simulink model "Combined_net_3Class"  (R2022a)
settings: Solver=FixedStepAuto  StartTime=0.0  StopTime=simtime  FixedStep=1  RelTol=1e-3
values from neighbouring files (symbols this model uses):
  simtime = length(SOC_CC{1, 1})    [Data_preparation.m]    (also in SimulationCycle.m = cell2mat(simtime_og(i)))
  SOH_predict = double(ans.SOHout(simtime))    [SimulationCycle.m]
undefined symbols (not defined in the file or in its folder): dSOC_mu_CC, dSOC_sig_CC, dv_mu_CC, dv_sig_CC, SOC_mu_CC, SOC_sig_CC, SOE_mu_CC, SOE_sig_CC
libraries: neural x121, deeplib x1
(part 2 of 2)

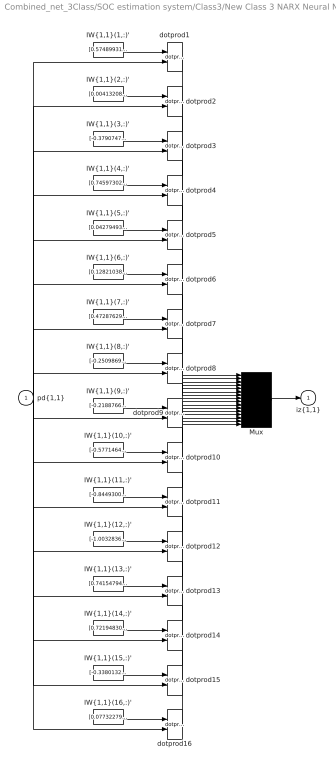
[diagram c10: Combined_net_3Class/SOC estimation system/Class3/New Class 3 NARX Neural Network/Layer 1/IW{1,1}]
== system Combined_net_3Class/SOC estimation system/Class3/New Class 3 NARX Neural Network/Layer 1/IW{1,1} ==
  "pd{1,1}" : Inport  PortDimensions=6  SampleTime=1
  "IW{1,1}(1,:)'" : Constant  Value=[0.57489931629684110081512926626601256430149078369140625;-0.3515011151766405106400270597077906131744384765625;-0.235240138064670478712514523067511618137359619140625;-0.415665695112699740132455872299033217132091522216796875;-0.54083277905494309134581953912856988608837127685546875;0.2491902947301962989445911489383433945477008819580078125]
  "IW{1,1}(10,:)'" : Constant  Value=[-0.57714648597659190532027650988311506807804107666015625;0.047702980401234530705156799967880942858755588531494140625;0.438905821704081822165477433372871018946170806884765625;0.5136719729138483625519029374117963016033172607421875;-0.06710567452929290521712601957915467210114002227783203125;-0.451124189798159325182069778747973032295703887939453125]
  "IW{1,1}(11,:)'" : Constant  Value=[-0.84493007670864195279847308484022505581378936767578125;0.0299673301415608085707109609074905165471136569976806640625;0.63504695757984752635394443132099695503711700439453125;-0.78817262284074451894611001989687792956829071044921875;0.91885523230133447913914324090001173317432403564453125;-0.8192881318045144301009941045776940882205963134765625]
  "IW{1,1}(12,:)'" : Constant  Value=[-1.00328365957425713617112705833278596401214599609375;-0.4162739419152441389115892889094538986682891845703125;0.2778056257659071714982701450935564935207366943359375;0.81259865037192724468440019336412660777568817138671875;1.23650985871420449058177837287075817584991455078125;-0.2929172509986999184405931373476050794124603271484375]
  "IW{1,1}(13,:)'" : Constant  Value=[0.74154794238423249463920683410833589732646942138671875;-0.48527842225931550057538288456271402537822723388671875;0.86708245679925510795982290801475755870342254638671875;-0.1759789359971944133764765183514100499451160430908203125;-1.3752493967582399836402373693999834358692169189453125;-0.00091260160326845523627581346914894311339594423770904541015625]
  "IW{1,1}(14,:)'" : Constant  Value=[0.72194830081038130487058879225514829158782958984375;0.083263215679716839900947888963855803012847900390625;0.768923477287991818940326993470080196857452392578125;0.1933662663322287811329402984483749605715274810791015625;1.308738303825084159370817360468208789825439453125;-0.57527297822178213859700690591125749051570892333984375]
  "IW{1,1}(15,:)'" : Constant  Value=[-0.338013217203540328181787799621815793216228485107421875;-0.11116352190086421780623737731730216182768344879150390625;-0.636515796112465448430839387583546340465545654296875;-1.03325458248108947856280792620964348316192626953125;1.334039636242204007743339388980530202388763427734375;0.93930340463265993289354582884698174893856048583984375]
  "IW{1,1}(16,:)'" : Constant  Value=[0.07732279602847856592173769740838906727731227874755859375;-0.406242406915276077494780793131212703883647918701171875;0.0246450504641358043855792203657983918674290180206298828125;-0.07305262802981961345327732715304591692984104156494140625;0.38838168508634407505297758689266629517078399658203125;-0.02468603065919001970929258504838799126446247100830078125]
  "IW{1,1}(2,:)'" : Constant  Value=[0.004132082293141054428475822390964822261594235897064208984375;-0.07626335722691372775994267385613056831061840057373046875;0.012693474527892857628419420734644518233835697174072265625;-0.0058209828312985149867397893785891938023269176483154296875;0.0780918658530748988066960691867279820144176483154296875;-0.01319417224404989714969804737165759433992207050323486328125]
  "IW{1,1}(3,:)'" : Constant  Value=[-0.379074783991779185043924371711909770965576171875;1.016745025307583372153885648003779351711273193359375;-0.442564886903998366829426913682254962623119354248046875;0.93193801751100113772707800308126024901866912841796875;-0.54900708871000547528495872029452584683895111083984375;0.56770819572392994256659903840045444667339324951171875]
  "IW{1,1}(4,:)'" : Constant  Value=[0.745973028967485074502974384813569486141204833984375;0.76493541460268821285950480159954167902469635009765625;-0.68912609389738832543770286065409891307353973388671875;0.07391887270039194934856396912437048740684986114501953125;0.81792600024676165304526875843293964862823486328125;0.27949425616045697751133047859184443950653076171875]
  "IW{1,1}(5,:)'" : Constant  Value=[0.04279493192384183075649417560271103866398334503173828125;-0.24990879501025708986361451025004498660564422607421875;0.008266010129701496789156323075076215900480747222900390625;-0.03680818383380424219097903915098868310451507568359375;0.225757554997183917944170161717920564115047454833984375;-0.008529510970860222640599346277667791582643985748291015625]
  "IW{1,1}(6,:)'" : Constant  Value=[0.12821038490724101510664922898286022245883941650390625;-0.58355828505747309176143744480214081704616546630859375;0.005953497815920946560630522270685105468146502971649169921875;-0.111167669930111123743898815519060008227825164794921875;0.52302756879668221845491871135891415178775787353515625;-0.00612713488324014531050121235011829412542283535003662109375]
  "IW{1,1}(7,:)'" : Constant  Value=[0.472876296890176905929337181078153662383556365966796875;0.507349771020651818531632670783437788486480712890625;0.4316557440097958942004652271862141788005828857421875;-0.58380532843848154112009751770528964698314666748046875;-0.0755903965904468899683621430085622705519199371337890625;-0.447270650721935447702293231486692093312740325927734375]
  "IW{1,1}(8,:)'" : Constant  Value=[-0.2509869071349084546085350666544400155544281005859375;0.341748594182761544768567318897112272679805755615234375;-0.6811569018579881618080662519787438213825225830078125;-0.98272991511463125835490473036770708858966827392578125;-0.82930046363700693490272897179238498210906982421875;0.60682317912345029586873579319217242300510406494140625]
  "IW{1,1}(9,:)'" : Constant  Value=[-0.2188766968978141658208613762326422147452831268310546875;-0.4951250680687657723666461606626398861408233642578125;-0.3781747939072890307699026379850693047046661376953125;0.51581894069656220036534932660288177430629730224609375;-0.53936529448250791762831113373977132141590118408203125;0.348952666019013424403283352148719131946563720703125]
  Mux : Mux  Inputs=16
  dotprod{1..16} (16 alike) : neural/Weight Functions/dotprod
  "iz{1,1}" : Outport
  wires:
  "IW{1,1}(1,:)'"/1 -> dotprod1/1
  "pd{1,1}"/1 -> dotprod1/2, dotprod2/2, dotprod3/2, dotprod4/2, dotprod5/2, dotprod6/2, dotprod7/2, dotprod8/2, dotprod9/2, dotprod10/2, dotprod11/2, dotprod12/2, dotprod13/2, dotprod14/2, dotprod15/2, dotprod16/2
  dotprod1/1 -> Mux/1
  "IW{1,1}(2,:)'"/1 -> dotprod2/1
  dotprod2/1 -> Mux/2
  "IW{1,1}(3,:)'"/1 -> dotprod3/1
  dotprod3/1 -> Mux/3
  "IW{1,1}(4,:)'"/1 -> dotprod4/1
  dotprod4/1 -> Mux/4
  "IW{1,1}(5,:)'"/1 -> dotprod5/1
  dotprod5/1 -> Mux/5
  "IW{1,1}(6,:)'"/1 -> dotprod6/1
  dotprod6/1 -> Mux/6
  "IW{1,1}(7,:)'"/1 -> dotprod7/1
  dotprod7/1 -> Mux/7
  "IW{1,1}(8,:)'"/1 -> dotprod8/1
  dotprod8/1 -> Mux/8
  "IW{1,1}(9,:)'"/1 -> dotprod9/1
  dotprod9/1 -> Mux/9
  "IW{1,1}(10,:)'"/1 -> dotprod10/1
  dotprod10/1 -> Mux/10
  "IW{1,1}(11,:)'"/1 -> dotprod11/1
  dotprod11/1 -> Mux/11
  "IW{1,1}(12,:)'"/1 -> dotprod12/1
  dotprod12/1 -> Mux/12
  "IW{1,1}(13,:)'"/1 -> dotprod13/1
  dotprod13/1 -> Mux/13
  "IW{1,1}(14,:)'"/1 -> dotprod14/1
  dotprod14/1 -> Mux/14
  "IW{1,1}(15,:)'"/1 -> dotprod15/1
  dotprod15/1 -> Mux/15
  "IW{1,1}(16,:)'"/1 -> dotprod16/1
  dotprod16/1 -> Mux/16
  Mux/1 -> "iz{1,1}"/1

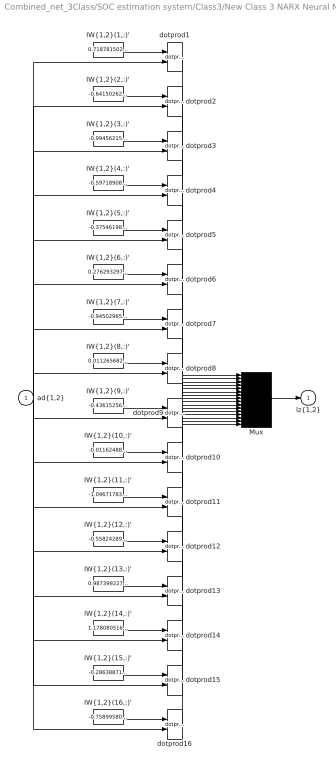
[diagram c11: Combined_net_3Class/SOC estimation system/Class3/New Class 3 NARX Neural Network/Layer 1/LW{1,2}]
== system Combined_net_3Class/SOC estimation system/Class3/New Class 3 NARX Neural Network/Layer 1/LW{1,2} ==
  "ad{1,2}" : Inport  PortDimensions=1  SampleTime=1
  "IW{1,2}(1,:)'" : Constant  Value=0.71878150211169489214313443881110288202762603759765625
  "IW{1,2}(10,:)'" : Constant  Value=-0.01162488589042467122813828694916082895360887050628662109375
  "IW{1,2}(11,:)'" : Constant  Value=-1.0967178319018591192701705949730239808559417724609375
  "IW{1,2}(12,:)'" : Constant  Value=-0.55824289911548652387551783249364234507083892822265625
  "IW{1,2}(13,:)'" : Constant  Value=0.9873992270040805596664768017944879829883575439453125
  "IW{1,2}(14,:)'" : Constant  Value=1.1780805168430548146574210477410815656185150146484375
  "IW{1,2}(15,:)'" : Constant  Value=-0.28638871201418203416011465378687717020511627197265625
  "IW{1,2}(16,:)'" : Constant  Value=-0.758995805205835427642568902228958904743194580078125
  "IW{1,2}(2,:)'" : Constant  Value=-0.64150262074499320164022719836793839931488037109375
  "IW{1,2}(3,:)'" : Constant  Value=-0.9945621582289432272006024504662491381168365478515625
  "IW{1,2}(4,:)'" : Constant  Value=-0.59718908368235179562333314606803469359874725341796875
  "IW{1,2}(5,:)'" : Constant  Value=-0.37546198082295989539858283023932017385959625244140625
  "IW{1,2}(6,:)'" : Constant  Value=0.276293297318553732200285821818397380411624908447265625
  "IW{1,2}(7,:)'" : Constant  Value=-0.9450296512095632817107571099768392741680145263671875
  "IW{1,2}(8,:)'" : Constant  Value=0.01126568217795320507590428604771659593097865581512451171875
  "IW{1,2}(9,:)'" : Constant  Value=-0.436152569616356677872914815452531911432743072509765625
  Mux : Mux  Inputs=16
  dotprod{1..16} (16 alike) : neural/Weight Functions/dotprod
  "lz{1,2}" : Outport
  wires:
  "IW{1,2}(1,:)'"/1 -> dotprod1/1
  "ad{1,2}"/1 -> dotprod1/2, dotprod2/2, dotprod3/2, dotprod4/2, dotprod5/2, dotprod6/2, dotprod7/2, dotprod8/2, dotprod9/2, dotprod10/2, dotprod11/2, dotprod12/2, dotprod13/2, dotprod14/2, dotprod15/2, dotprod16/2
  dotprod1/1 -> Mux/1
  "IW{1,2}(2,:)'"/1 -> dotprod2/1
  dotprod2/1 -> Mux/2
  "IW{1,2}(3,:)'"/1 -> dotprod3/1
  dotprod3/1 -> Mux/3
  "IW{1,2}(4,:)'"/1 -> dotprod4/1
  dotprod4/1 -> Mux/4
  "IW{1,2}(5,:)'"/1 -> dotprod5/1
  dotprod5/1 -> Mux/5
  "IW{1,2}(6,:)'"/1 -> dotprod6/1
  dotprod6/1 -> Mux/6
  "IW{1,2}(7,:)'"/1 -> dotprod7/1
  dotprod7/1 -> Mux/7
  "IW{1,2}(8,:)'"/1 -> dotprod8/1
  dotprod8/1 -> Mux/8
  "IW{1,2}(9,:)'"/1 -> dotprod9/1
  dotprod9/1 -> Mux/9
  "IW{1,2}(10,:)'"/1 -> dotprod10/1
  dotprod10/1 -> Mux/10
  "IW{1,2}(11,:)'"/1 -> dotprod11/1
  dotprod11/1 -> Mux/11
  "IW{1,2}(12,:)'"/1 -> dotprod12/1
  dotprod12/1 -> Mux/12
  "IW{1,2}(13,:)'"/1 -> dotprod13/1
  dotprod13/1 -> Mux/13
  "IW{1,2}(14,:)'"/1 -> dotprod14/1
  dotprod14/1 -> Mux/14
  "IW{1,2}(15,:)'"/1 -> dotprod15/1
  dotprod15/1 -> Mux/15
  "IW{1,2}(16,:)'"/1 -> dotprod16/1
  dotprod16/1 -> Mux/16
  Mux/1 -> "lz{1,2}"/1

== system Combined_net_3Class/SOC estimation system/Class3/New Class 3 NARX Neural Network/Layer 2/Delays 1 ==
  "p{2}" : Inport  PortDimensions=16  SampleTime=1
  mux : Mux  Inputs=1
  "pd{2,1}" : Outport
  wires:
  "p{2}"/1 -> mux/1
  mux/1 -> "pd{2,1}"/1

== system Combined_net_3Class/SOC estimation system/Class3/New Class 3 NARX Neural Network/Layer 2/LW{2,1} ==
  "ad{2,1}" : Inport  PortDimensions=16  SampleTime=1
  "IW{2,1}(1,:)'" : Constant  Value=[-0.328969104320398830765270759002305567264556884765625;-0.69040742906918894927770224967389367520809173583984375;-0.0004795505652991080623552544448529033616068772971630096435546875;2.46859355071712459144504803187913921647123061120510101318359375e-05;-1.66117477546487268824648708687163889408111572265625;0.8123379487254569486509581111022271215915679931640625;-0.00225935989402721235097537544334045378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
  Mux : Mux  Inputs=1
  dotprod1 : neural/Weight Functions/dotprod
  "lz{2,1}" : Outport
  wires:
  "IW{2,1}(1,:)'"/1 -> dotprod1/1
  "ad{2,1}"/1 -> dotprod1/2
  dotprod1/1 -> Mux/1
  Mux/1 -> "lz{2,1}"/1

== matlab function Combined_net_3Class/If Action
Subsystem/SOH estimation system/Subsystem1/MATLAB Function ==
function dV  = V_features(V_03,dv_mu_CC,dv_sig_CC)
dV = ((V_03(120-11)-V_03(1+10))-dv_mu_CC)/dv_sig_CC;
% if dV<-5 || dV>1
%     dV = 0;
% end
end

== matlab function Combined_net_3Class/If Action
Subsystem/SOH estimation system/Subsystem1/MATLAB Function1 ==
function SOE  = SOE(I_03,V_03,SOE_mu_CC,SOE_sig_CC)

persistent  E1 E2 E3 E4 dE flag1 flag2 count SOE_reg
if isempty(E1)
    E1 = 0;
    E2 = 0;
    E3 = 0;
    E4 = 0;
    dE = 0;
    flag1 = 0;
    flag2 = 1;
    count = 0;
    SOE_reg = 0;
end

if I_03 ~= 0
    count = count+1;
end

if I_03(1)~=0 && flag1 ==0 && flag2 == 1
    E1 = I_03(1)*V_03(1);
    E2 = I_03(120)*V_03(120);
    flag1 = 1;
    flag2 = 0;
elseif I_03(1)~=0 && flag1 == 1 && flag2 == 0
    E3 = I_03(1)*V_03(1);
    E4 = I_03(120)*V_03(120);
    flag1 = 0;
    flag2 = 1;
end

SOE1 = zeros(1,120);

if count == 1
    SOE1(1) = 0;
elseif mod(count,2) == 1
    dE = (E1-E4)/2;
    SOE1(1) = SOE_reg+dE;
else
    dE = (E3-E2)/2;
    SOE1(1) = SOE_reg+dE;
end

time = linspace(1,120,120);
E = I_03.*V_03;
SOE_cum = cumtrapz(time,E);
k = 2;

for i = 1:119
    SOE1(k) = SOE_cum(i+1)-SOE_cum(i);
    k = k+1;
end

SOE_reg = SOE1(120);

SOE = (SOE1(120-11)-SOE_mu_CC)/SOE_sig_CC;
end

== matlab function Combined_net_3Class/If Action
Subsystem/SOH estimation system/Subsystem1/MATLAB Function2 ==
function [SOC,dSOC] = SOC_features(SOC_03,SOC_mu_CC,SOC_sig_CC,dSOC_mu_CC,dSOC_sig_CC)
SOC = (SOC_03(120-11)-SOC_mu_CC)/SOC_sig_CC;
dSOC = ((SOC_03(120-11)-SOC_03(1+10))-dSOC_mu_CC)/dSOC_sig_CC;
if dSOC<-10
    dSOC = 0;
end
end

== matlab function Combined_net_3Class/If Action
Subsystem/SOH estimation system/Subsystem1/MOVMEAN ==
function V_filt = filt(V)

V_filt = movmean(V,10);


end

== matlab function Combined_net_3Class/If Action
Subsystem/SOH estimation system/Subsystem1/MOVMEAN1 ==
function I_filt = filt(I)

I_filt = movmean(I,10);


end
